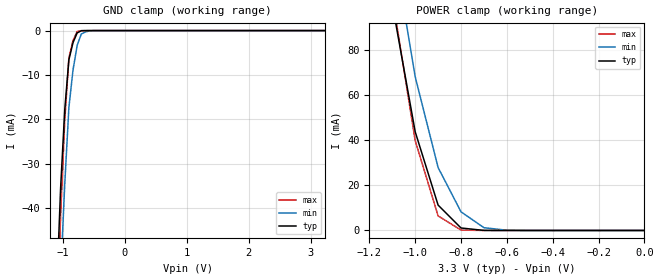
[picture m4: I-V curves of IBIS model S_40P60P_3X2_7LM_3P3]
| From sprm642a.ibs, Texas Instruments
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|IQ0442FS_40P60P_3X2_PD_3P3; PULLDOWN_ON
|   Model Cell S_40P60P_3X2_7LM_3P3
|IQ0442FS_40P60P_3X2_3P3
[Model]   S_40P60P_3X2_7LM_3P3
Model_type   Input
Polarity   Non-Inverting
Vinl =  1.55
Vinh =  1.75
C_comp   1.2p   1.2p   1.2p
[Model Spec]
Vinl   1.55   1.42   1.68
Vinh   1.75   1.55   1.85
[Temperature Range]   25   155   -40
[Voltage Range]   3.3   2.97   3.63
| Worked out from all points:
|   GND clamp passes 1 mA (typ) near -0.78 V on its own axis
|   POWER clamp passes 1 mA (typ) near -0.79 V on its own axis
[POWER_clamp]
|   voltage   I(typ)   I(min)   I(max)
-3.3V     1.823A     2.351A     1.96A
-1.1V     100.7mA    129.7mA    103.9mA
-1.067V   81.76mA    109.2mA    82.61mA
-1.033V   62.81mA    88.77mA    61.28mA
-1V       43.87mA    68.31mA    39.95mA
-900mV    11.27mA    27.96mA    6.481mA
-800mV    1.099mA    8.283mA    176.7uA
-700mV    35.91uA    1.232mA    3.424uA
-600mV    1.374uA    111.2uA    455.2nA
0V        175pA      247.2pA    192.5pA
[GND_clamp]
|   voltage   I(typ)   I(min)   I(max)
-3.3V     -1.38A     -1.323A    -2.074A
-1.1V     -59.59mA   -79.11mA   -70.71mA
-1.033V   -35.48mA   -55.25mA   -41.82mA
-966.7mV  -17.81mA   -34.65mA   -20.29mA
-900mV    -6.579mA   -17.32mA   -6.122mA
-833.3mV  -2.708mA   -8.853mA   -2.234mA
-766.7mV  -527.2uA   -3.335mA   -196uA
-700mV    -37.17uA   -765.8uA   -8.209uA
-566.7mV  -1.613uA   -62.15uA   -984.8nA
3.233V    169pA      53.88nA    156.8pA
